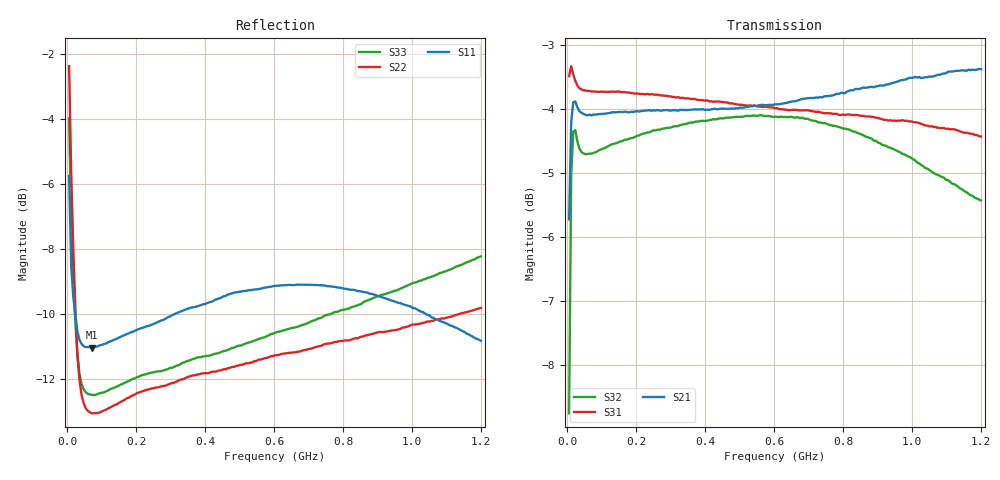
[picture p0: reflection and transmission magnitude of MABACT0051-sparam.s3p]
#	MHz	S	RI	R	75
!FREQ	R1	I1	R2	I2	R3	I3
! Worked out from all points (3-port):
!   201 points, 5 MHz to 1.2 GHz, reference 75 ohm
!   strongest paths, dB at 5 MHz, 303.8 MHz, 602.5 MHz, 901.2 MHz, 1.2 GHz:
!     S21: -5.7, -4.0, -3.9, -3.6, -3.4
!     S31: -3.5, -3.8, -4.0, -4.1, -4.4
!     S32: -8.8, -4.3, -4.1, -4.5, -5.4
!   lowest |S11| = -11.0 dB at 70.72 MHz (marker M1), VSWR 1.78, Z = 132 - j12.9 ohm
!   |S11| at or under -10 dB: 22.51 MHz to 312.5 MHz (290 MHz wide, 173 % of centre); 1.04 GHz to end of sweep
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5  0.0712 0.5101  -0.4413 -0.272  0.6279 0.2311
   -0.4388 -0.2735  -0.4349 0.6228  0.127 0.3444
   0.6279 0.2311  0.1239 0.343  -0.252 0.5799
10.975  0.2715 0.2578  -0.5916 -0.1712  0.6771 0.0753
        -0.5908 -0.1711  0.0402 0.5219  0.4472 0.3371
        0.6771 0.0753  0.4454 0.3376  0.1196 0.4236
16.95  0.3043 0.1443  -0.6308 -0.1002  0.671 0.0277
       -0.6305 -0.1003  0.1941 0.3515  0.5599 0.2328
       0.671 0.0277  0.5587 0.2335  0.2274 0.2772
22.925  0.3046 0.0791  -0.6377 -0.0528  0.6635 0.00397
        -0.6372 -0.0526  0.2304 0.2295  0.5887 0.1524
        0.6635 0.00397  0.5876 0.1526  0.2504 0.179
34.875  0.2876 0.0229  -0.6282 -0.00772  0.6544 -0.0196
        -0.6282 -0.00674  0.2161 0.1275  0.5816 0.0835
        0.6544 -0.0196  0.5814 0.0836  0.237 0.0969
70.725  0.277 -0.0452  -0.6219 0.0506  0.6476 -0.064
        -0.6213 0.0499  0.2155 0.0551  0.5812 0.0348
        0.6476 -0.064  0.581 0.0354  0.2352 0.0338
339.6  0.0903 -0.3076  -0.5336 0.3356  0.5526 -0.3287
       -0.5337 0.3338  0.2217 -0.1185  0.6075 -0.0887
       0.5526 -0.3287  0.6073 -0.0882  0.2273 -0.1388
602.5  -0.1844 -0.2965  -0.3478 0.5335  0.3659 -0.5148
       -0.3506 0.5307  0.169 -0.2145  0.5877 -0.2061
       0.3659 -0.5148  0.5874 -0.2049  0.168 -0.2433
895.275  -0.3326 -0.0601  -0.072 0.6507  0.0844 -0.6153
         -0.077 0.6524  0.1052 -0.2764  0.5075 -0.312
         0.0844 -0.6153  0.5078 -0.3112  0.0886 -0.3238
1200  -0.2047 0.2018  0.2481 0.6239  -0.2352 -0.5522
      0.248 0.6305  0.041 -0.3203  0.4095 -0.3454
      -0.2352 -0.5522  0.4091 -0.3447  -0.0109 -0.3873
